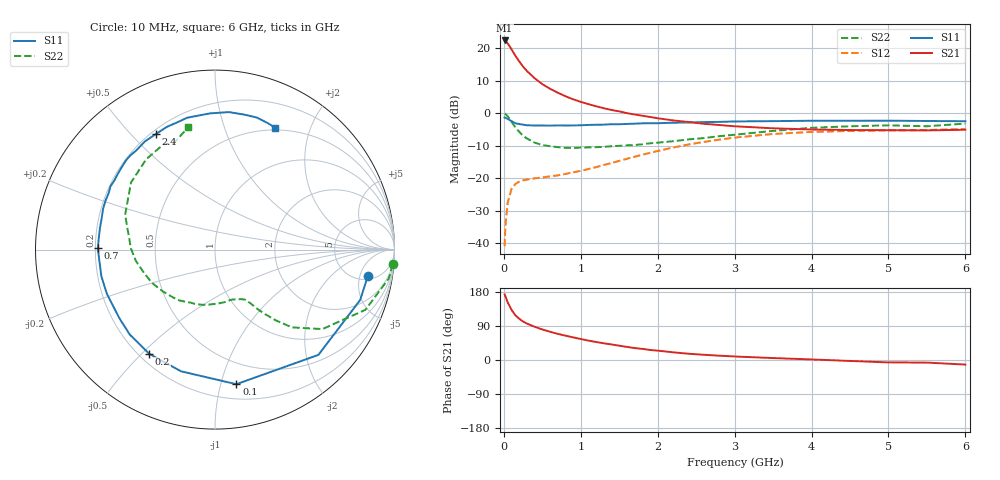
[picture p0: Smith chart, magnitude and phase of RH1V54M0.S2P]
! SIEMENS Small Signal Semiconductors
! BFR106
! Si NPN RF Bipolar Junction Transistor in SOT23
! VCE = 1.5 V  IC = 4 mA
! Common Emitter S-Parameters:  August  1996
# GHz  S  MA  R  50
!  f  S11  S21  S12  S22
! GHz  MAG  ANG  MAG  ANG  MAG  ANG  MAG  ANG
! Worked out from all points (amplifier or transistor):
!   36 points, 10 MHz to 6 GHz, reference 50 ohm
!   highest |S21| = 22.5 dB at 10 MHz (marker M1)
!   |S21| within 3 dB of that: start of sweep to 107.1 MHz
!   unconditionally stable (mu >= 1): 650.7 MHz to 2.348 GHz; 3.631 GHz to end of sweep
!   at 250 MHz: K = 0.45, MSG = 17.5 dB, |S12| = -20.6 dB
!   at 1.4 GHz: K = 1.19, MAG = 5.5 dB, |S12| = -15.3 dB
!   at 6 GHz: K = 1.03, MAG = -1.1 dB, |S12| = -4.8 dB
!   S11 on the Smith chart (normalised r, x): 10 MHz: 5.87, -6.74; 100 MHz: 0.32, -1.12; 200 MHz: 0.24, -0.53; 700 MHz: 0.21, +0.01; 2.4 GHz: 0.22, +0.59; 6 GHz: 0.47, +1.51
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0.01  0.8641 -9.7  13.29 173.4  0.009 85.7  0.9924 -4.7
0.02  0.8563 -19.1  13.14 168.5  0.0183 78.6  0.9819 -9.4
0.05  0.8222 -45.5  11.97 152.0  0.0421 66.3  0.9028 -21.8
0.1  0.7593 -81.0  9.718 132.4  0.0684 50.9  0.7444 -36.5
0.15  0.704 -105.6  7.72 117.9  0.0817 40.9  0.6098 -45.3
0.2  0.6866 -122.3  6.318 108.9  0.0889 36.3  0.5206 -49.3
0.25  0.6704 -135.1  5.253 101.5  0.0929 32.9  0.4523 -52.3
0.3  0.6559 -144.2  4.495 96.2  0.0955 31.9  0.4106 -54.3
0.4  0.6509 -157.7  3.482 87.7  0.0998 31.3  0.3541 -56.8
0.5  0.6503 -166.7  2.822 80.6  0.103 32.5  0.3253 -59.0
0.6  0.6475 -174.7  2.395 74.6  0.1072 34.7  0.312 -62.2
0.7  0.6528 179.2  2.085 69.0  0.1109 37.4  0.3022 -66.2
0.9  0.6523 169.2  1.649 59.7  0.1234 43.1  0.2936 -73.8
1.1  0.6637 160.0  1.387 51.2  0.139 48.1  0.2993 -83.6
1.6  0.6872 141.7  1.008 34.6  0.1999 54.7  0.3219 -109.3
2.2  0.7183 122.9  0.779 20.3  0.2976 51.5  0.3722 -141.1
2.4  0.7233 117.0  0.737 16.5  0.3316 48.6  0.3973 -152.2
3.5  0.7594 92.1  0.589 5.1  0.4818 28.2  0.5371 158.8
4.5  0.7696 77.6  0.554 -2.5  0.5356 10.3  0.6328 127.2
5  0.7718 72.3  0.551 -6.4  0.5457 3.3  0.6547 115.6
5.5  0.7633 67.2  0.546 -6.8  0.5537 0.0  0.6328 111.9
6  0.7571 63.6  0.56 -12.1  0.5757 -7.2  0.6967 102.4
